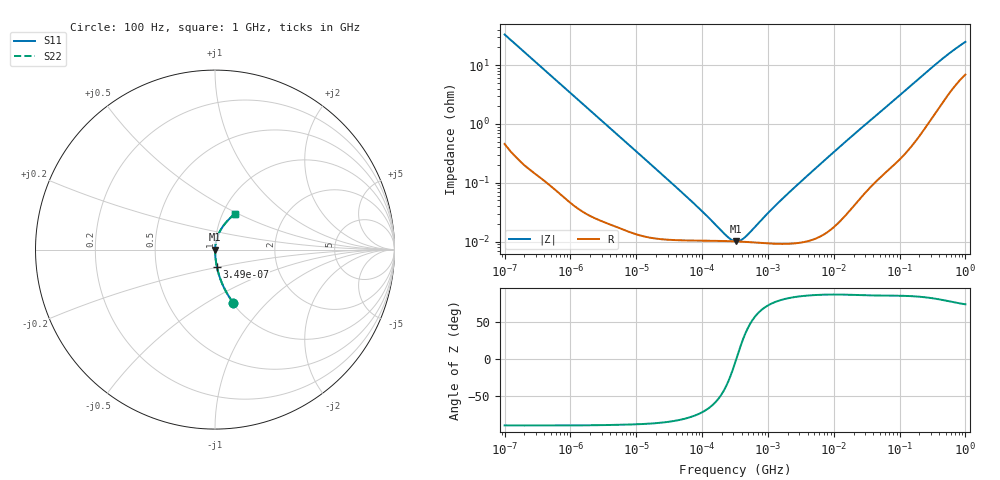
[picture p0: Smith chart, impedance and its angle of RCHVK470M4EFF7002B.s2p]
! RCHVK470M4EFF7002B  S-PARAMETER MODEL  (AEC-Q200 qualified)
! Model Generated by ELNA Corporation (http://www.ty-top.com)
! Version 1.0
! ELNA Control No. 240315
! Copyright (c) 2024 ELNA CO.,LTD. All Rights Reserved.
! Products Name : CONDUCTIVE POLYMER HYBRID ALUMINUM ELECTROLYTIC CAPACITORS
! Characteristics :
!  Capacitance  :  47uF  ,  Rated voltage  :  63V
!  Operating Temp. Range  :  -55 to +125 degC  ,  Endurance  :  6000hr at 125 degC
!  Dimension D  :  10mm  ,  Dimension L  :  8.7mm
! Frequency Range : 100Hz - 1GHz
! External Node Assignments :
!  1  o---| |---o  2
# MHz S RI R 50
!Freq[MHz].  S11 Real  S11 Imag  S21 Real  S21 Imag  S12 Real  S12 Imag  S22 Real  S22 Imag
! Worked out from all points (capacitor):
!   401 points, 100 Hz to 1 GHz, reference 50 ohm
!   read as one part in series: C = 48 uF near 108 Hz
!   lowest |Z| = 10.1 mohm at 329.2 kHz (marker M1)
!   series resonance near 330.5 kHz, so ESL is about 4.8 nH
!   S11 on the Smith chart (normalised r, x): 100 Hz: 1.01, -0.66; 349 Hz: 1.00, -0.19; 1 GHz: 1.14, +0.48
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0.0001  0.1022 -0.2961  0.8978 0.2961  0.8978 0.2961  0.1022 -0.2961
0.000113  0.0824 -0.2685  0.9176 0.2685  0.9176 0.2685  0.0824 -0.2685
0.000176  0.0364 -0.1815  0.9636 0.1815  0.9636 0.1815  0.0364 -0.1815
0.000349  0.0102 -0.0944  0.9898 0.0944  0.9898 0.0944  0.0102 -0.0944
0.000638  0.00344 -0.0522  0.9966 0.0522  0.9966 0.0522  0.00344 -0.0522
0.001488  0.00084 -0.0226  0.9992 0.0226  0.9992 0.0226  0.00084 -0.0226
0.022131  0.000113 -0.00154  0.9999 0.00154  0.9999 0.00154  0.000113 -0.00154
0.087096  0.000104 -0.000366  0.9999 0.000366  0.9999 0.000366  0.000104 -0.000366
0.238506  0.000102 -6.93e-05  0.9999 6.93e-05  0.9999 6.93e-05  0.000102 -6.93e-05
0.280221  0.000102 -3.47e-05  0.9999 3.47e-05  0.9999 3.47e-05  0.000102 -3.47e-05
0.316228  0.000101 -9.25e-06  0.9999 9.25e-06  0.9999 9.25e-06  0.000101 -9.25e-06
0.32923  0.000101 -8.03e-07  0.9999 8.03e-07  0.9999 8.03e-07  0.000101 -8.03e-07
0.386812  0.0001 3.32e-05  0.9999 -3.32e-05  0.9999 -3.32e-05  0.0001 3.32e-05
0.473151  9.88e-05 7.75e-05  0.9999 -7.75e-05  0.9999 -7.75e-05  9.88e-05 7.75e-05
1.348963  9.19e-05 0.000418  0.9999 -0.000418  0.9999 -0.000418  9.19e-05 0.000418
4.704354  0.000109 0.00156  0.9999 -0.00156  0.9999 -0.00156  0.000109 0.00156
17.78279  0.000377 0.00584  0.9996 -0.00584  0.9996 -0.00584  0.000377 0.00584
69.9842  0.00216 0.0215  0.9978 -0.0215  0.9978 -0.0215  0.00216 0.0215
176.8072  0.00789 0.0522  0.9921 -0.0522  0.9921 -0.0522  0.00789 0.0522
395.8221  0.0303 0.1075  0.9697 -0.1075  0.9697 -0.1075  0.0303 0.1075
668.3439  0.0669 0.1578  0.9331 -0.1578  0.9331 -0.1578  0.0669 0.1578
1000  0.109 0.1989  0.891 -0.1989  0.891 -0.1989  0.109 0.1989
